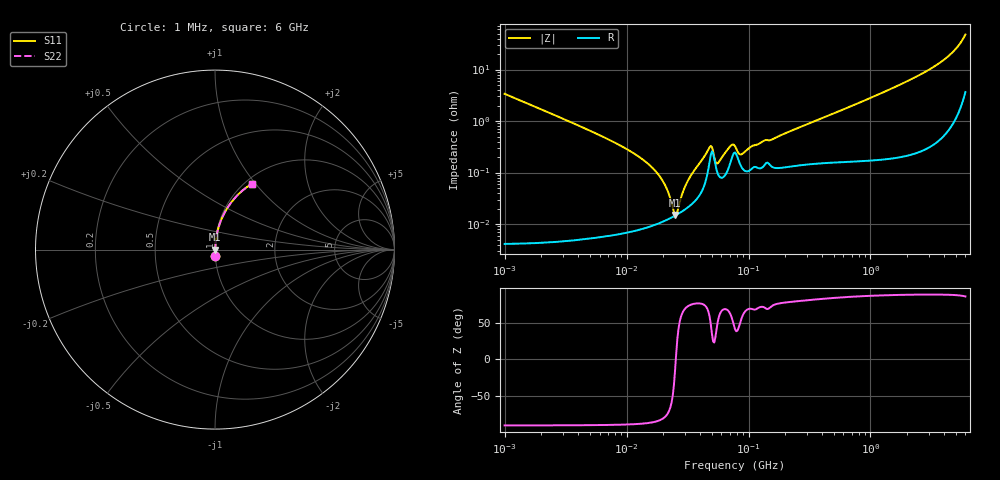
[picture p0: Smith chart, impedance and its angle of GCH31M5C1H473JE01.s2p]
!Murata Part Number: GCH31M5C1H473JE01
!These Parameters are Measured in Series Mode Connection
!Data Generated on Mar 13, 2026
!  o--ll--o
!Port1  Port2
!  o------o
!Operation Temp=25[degC], DC Bias Voltage=0[V]
!Freq. Start=1000[kHz] Stop=6[GHz] 401[Steps]
# Hz S RI R 50
!Freq.(Hz) S11(Real) S11(Imag) S21(Real) S21(Imag) S12(Real) S12(Imag) S22(Real) S22(Imag)
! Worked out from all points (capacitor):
!   401 points, 1 MHz to 6 GHz, reference 50 ohm
!   read as one part in series: C = 47 nF near 1.044 MHz
!   lowest |Z| = 15.1 mohm at 25 MHz (marker M1)
!   series resonance near 25.34 MHz, so ESL is about 840 pH
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1000000  0.00118 -0.0338  0.9988 0.0338  0.9988 0.0338  0.00118 -0.0338
4293785  0.000109 -0.00766  0.9999 0.00766  0.9999 0.00766  0.000109 -0.00766
1.142569e7  7.84e-05 -0.00237  0.9999 0.00237  0.9999 0.00237  7.84e-05 -0.00237
1.843659e7  0.000104 -0.000878  0.9999 0.000878  0.9999 0.000878  0.000104 -0.000878
2.146833e7  0.000121 -0.000456  0.9999 0.000456  0.9999 0.000456  0.000121 -0.000456
2.499862e7  0.000146 -3.72e-05  0.9999 3.72e-05  0.9999 3.72e-05  0.000146 -3.72e-05
2.610999e7  0.000155 8.38e-05  0.9998 -8.38e-05  0.9998 -8.38e-05  0.000155 8.38e-05
2.910942e7  0.000182 0.000394  0.9998 -0.000394  0.9998 -0.000394  0.000182 0.000394
3.175522e7  0.000211 0.000656  0.9998 -0.000656  0.9998 -0.000656  0.000211 0.000656
4.800399e7  0.00166 0.00263  0.9983 -0.00263  0.9983 -0.00263  0.00166 0.00263
5.013812e7  0.00258 0.00178  0.9974 -0.00178  0.9974 -0.00178  0.00258 0.00178
5.351853e7  0.0014 0.000816  0.9986 -0.000816  0.9986 -0.000816  0.0014 0.000816
5.589783e7  0.000955 0.00117  0.999 -0.00117  0.999 -0.00117  0.000955 0.00117
7.100585e7  0.00156 0.00286  0.9984 -0.00286  0.9984 -0.00286  0.00156 0.00286
7.745967e7  0.00245 0.00214  0.9976 -0.00214  0.9976 -0.00214  0.00245 0.00214
8.825674e7  0.00124 0.00192  0.9988 -0.00192  0.9988 -0.00192  0.00124 0.00192
1.073387e8  0.00122 0.00305  0.9988 -0.00305  0.9988 -0.00305  0.00122 0.00305
3.325952e8  0.00155 0.00934  0.9985 -0.00934  0.9985 -0.00934  0.00155 0.00934
1.428092e9  0.0035 0.0406  0.9965 -0.0406  0.9965 -0.0406  0.0035 0.0406
3.638376e9  0.0209 0.128  0.9791 -0.128  0.9791 -0.128  0.0209 0.128
4.93336e9  0.0641 0.2244  0.9359 -0.2244  0.9359 -0.2244  0.0641 0.2244
6e9  0.2044 0.3667  0.7956 -0.3667  0.7956 -0.3667  0.2044 0.3667
